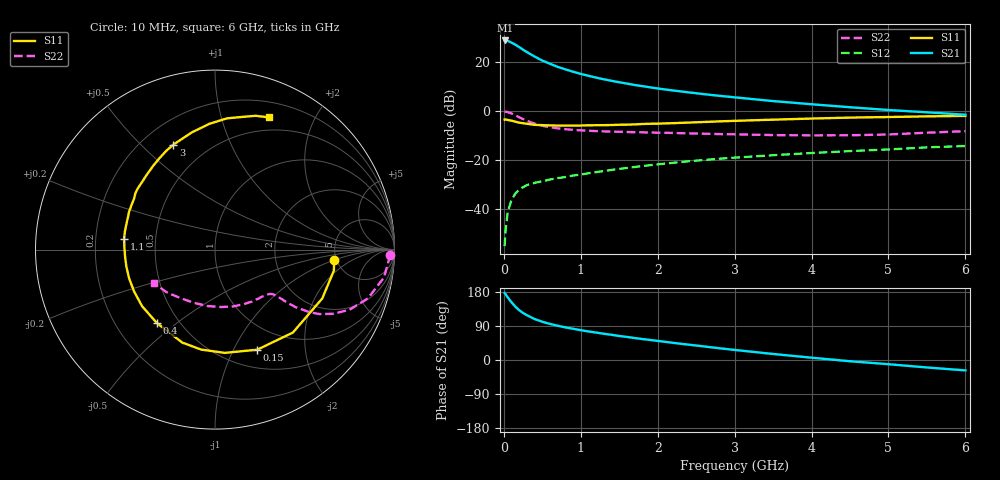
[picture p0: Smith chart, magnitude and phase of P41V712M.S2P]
! SIEMENS Small Signal Semiconductors
! BFP182
! Si NPN RF Bipolar Junction Transistor in SOT143
! VCE = 1.75 V  IC = 12 mA
! Common Emitter S-Parameters:  March  1996
# GHz  S  MA  R  50
!  f  S11  S21  S12  S22
! GHz  MAG  ANG  MAG  ANG  MAG  ANG  MAG  ANG
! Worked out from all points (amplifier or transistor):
!   36 points, 10 MHz to 6 GHz, reference 50 ohm
!   highest |S21| = 28.9 dB at 20 MHz (marker M1)
!   |S21| within 3 dB of that: start of sweep to 212.6 MHz
!   unconditionally stable (mu >= 1): 945.3 MHz to 5.402 GHz
!   at 250 MHz: K = 0.39, MSG = 28.2 dB, |S12| = -31.2 dB
!   at 1.4 GHz: K = 1.14, MAG = 16.0 dB, |S12| = -24.1 dB
!   at 6 GHz: K = 0.95, MSG = 6.4 dB, |S12| = -14.3 dB
!   S11 on the Smith chart (normalised r, x): 10 MHz: 4.77, -1.00; 150 MHz: 0.71, -1.25; 400 MHz: 0.38, -0.43; 1.1 GHz: 0.33, +0.05; 3 GHz: 0.32, +0.63; 6 GHz: 0.36, +1.43
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0.01  0.6662 -5.0  27.89 177.1  0.0017 81.6  0.9737 -1.7
0.02  0.6726 -10.0  27.99 174.5  0.0033 83.2  0.9694 -3.7
0.05  0.6566 -24.5  27.51 165.3  0.0084 82.8  0.954 -9.4
0.1  0.634 -46.8  25.27 152.2  0.0151 67.7  0.8941 -17.7
0.15  0.6053 -67.1  22.9 140.8  0.0205 60.9  0.8211 -24.1
0.2  0.578 -84.6  20.45 131.4  0.0247 55.3  0.7475 -28.6
0.25  0.5624 -97.9  18.06 123.9  0.0275 52.1  0.6837 -31.7
0.3  0.5491 -109.4  16.18 118.2  0.0304 49.7  0.6318 -33.5
0.4  0.5219 -128.4  13.09 108.1  0.0337 46.4  0.5521 -35.5
0.5  0.5142 -142.2  10.84 100.9  0.0364 44.9  0.4995 -36.3
0.6  0.5076 -152.7  9.312 95.2  0.0395 45.2  0.4651 -36.5
0.7  0.5046 -161.4  8.04 90.4  0.0422 45.0  0.4427 -36.8
0.9  0.5025 -175.5  6.402 82.4  0.0477 45.9  0.4116 -37.4
1.1  0.5106 173.2  5.282 75.3  0.0532 47.2  0.3944 -38.8
1.5  0.5236 156.0  3.891 63.4  0.0653 47.3  0.3764 -43.2
1.8  0.5425 145.0  3.242 55.3  0.0745 47.1  0.3664 -47.5
2.2  0.5644 132.3  2.638 45.3  0.0869 45.0  0.3557 -54.4
3  0.6293 111.6  1.911 26.6  0.1109 39.7  0.3332 -71.5
3.5  0.666 101.1  1.601 15.9  0.1244 35.8  0.3218 -84.0
4.5  0.7342 84.8  1.197 -3.3  0.1511 27.9  0.3189 -111.8
5.5  0.7786 73.2  0.942 -19.7  0.1802 20.1  0.36 -138.8
6  0.7954 67.9  0.84 -27.4  0.1918 15.3  0.387 -151.4
